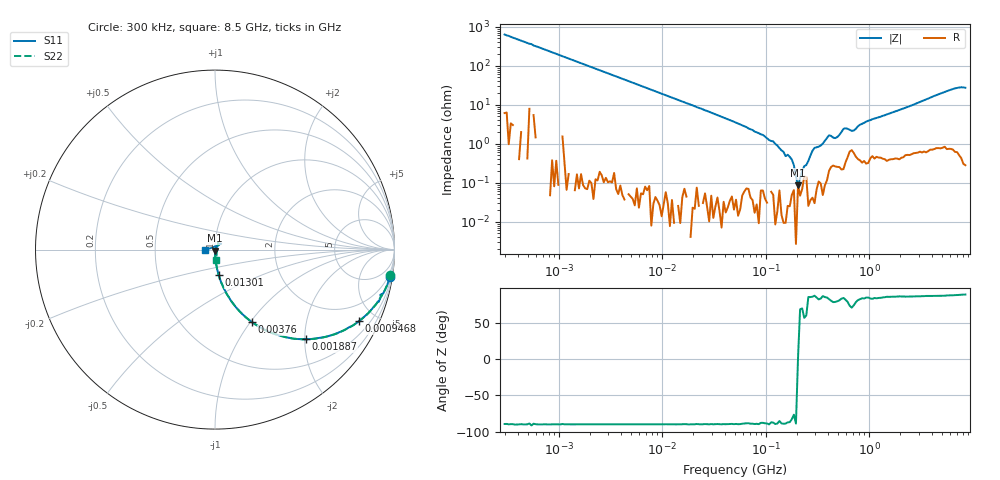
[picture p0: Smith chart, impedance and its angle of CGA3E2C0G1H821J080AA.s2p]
! S-parameter Generated by TDK Corporation
! Copyright(C) 2015 TDK Corporation.
! All Rights Reserved.
! TDK P/N: CGA3E2C0G1H821J080AA (Multilayer Ceramic Chip Capacitors)
! Property: C=820pF
! Size(LxWxT): 1.6x0.8x0.8mm, 0.063x0.031x0.031inches
! Model Type: s2p (Touchstone File Format Version 1.0)
! Frequency: DC=Yes Start=0.3MHz Stop=8500MHz 225points Log-sweep
! Note:
! Model Generated on Jun. 23, 2015
! Hash(MD5):
! Port Assignments:
!  1 ---| |--- 2
! Applicable Conditions:
!  Temperature = 25 degC
!  DC Bias Voltage = 0 V
!  Small Signal Operation
! Terms and conditions regarding TDK Simulation Models
! (1)This simulation model is being provided solely for informational purposes. Please refer to the specifications of the products in terms of detailed characteristics of such products.
! (2)In no event shall TDK Corporation of any of its subsidiaries be liable for any loss or damage arising, directly or indirectly,
!  From any information contained in this simulation model, including, but not limited to loss or damages arising from any inaccuracies, omissions or errors in connection with such information.
! (3)Any and all copyrights on this simulation model are owned by TDK Corporation.
!  Duplication or redistribution of this simulation model without prior written permission from TDK Corporation is prohibited.
! (4)This simulation model is subject to any modification or change without any prior notice.
! (5)Neither TDK Corporation nor any of its subsidiaries shall make any warranty, express or implied,
!  Including but not limited to the correctness, implied warranties of merchantability and fitness for a particular purpose with respect to this simulation models.
! (6)The use of this simulation model shall be deemed to have consented to the terms and conditions hereof.
# MHz S MA R 50
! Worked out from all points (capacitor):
!   224 points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, 300 kHz to 8.5 GHz, reference 50 ohm
!   read as one part in series: C = 834 pF near 314.1 kHz
!   lowest |Z| = 85 mohm at 205.2 MHz (marker M1)
!   series resonance near 205.1 MHz, so ESL is about 720 pH
!   S11 on the Smith chart (normalised r, x): 300 kHz: 1, -13; 946.8 kHz: 0.99, -4.02; 1.887 MHz: 1.00, -2.03; 3.76 MHz: 1.00, -1.02; 13.01 MHz: 1.00, -0.29; 8.5 GHz: 0.90, -0.00
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0.3  0.9867 -8.9  0.1558 80.8  0.1552 81.8  0.9877 -8.4
0.9467989  0.896 -26.5  0.444 63.5  0.4437 63.6  0.8957 -26.4
1.72111  0.7423 -42.0  0.669 48.0  0.6686 48.0  0.7431 -42.0
1.88686  0.7116 -44.6  0.7026 45.4  0.7026 45.4  0.7116 -44.6
3.760292  0.4532 -63.1  0.8905 26.9  0.8912 26.9  0.4532 -63.1
9.430415  0.1985 -78.5  0.98 11.4  0.9799 11.5  0.1984 -78.5
13.01035  0.1451 -81.7  0.9894 8.4  0.9891 8.3  0.1452 -81.6
51.67171  0.03639 -87.4  0.9991 1.9  0.9987 1.9  0.03628 -87.8
205.2186  0.005946 -85.1  0.9987 -0.3  0.9988 -0.4  0.006224 -87.3
283.1228  0.002287 -76.6  0.9996 -0.9  0.9993 -0.9  0.002069 -91.3
324.9909  0.001492 -54.3  0.9979 -1.0  0.9984 -1.0  0.0003405 -143.2
356.2888  0.001068 10.0  0.9999 -1.1  0.9988 -1.1  0.0009781 119.3
428.2171  0.003375 56.2  0.996 -1.6  0.9966 -1.6  0.003497 73.0
678.1388  0.007827 3.5  0.9925 -2.2  0.9927 -2.2  0.005203 24.2
778.4218  0.004203 1.3  0.9958 -3.2  0.9943 -3.1  0.002439 26.4
815.0429  0.002866 36.0  0.9962 -3.4  0.9964 -3.4  0.005513 14.5
1551.304  0.002911 56.3  0.9955 -6.6  0.9954 -6.6  0.005704 18.8
2240.89  0.002958 44.4  0.9947 -9.6  0.9929 -9.5  0.006532 -1.0
5619.915  0.04286 48.0  0.9912 -24.0  0.9901 -23.8  0.04276 64.3
7072.242  0.04326 47.1  0.9895 -30.0  0.9871 -29.9  0.04063 65.3
8118.083  0.01966 146.0  0.9911 -34.1  0.9909 -34.1  0.0193 -59.6
8500  0.0544 -178.1  0.989 -35.6  0.9911 -35.6  0.05821 -82.4
